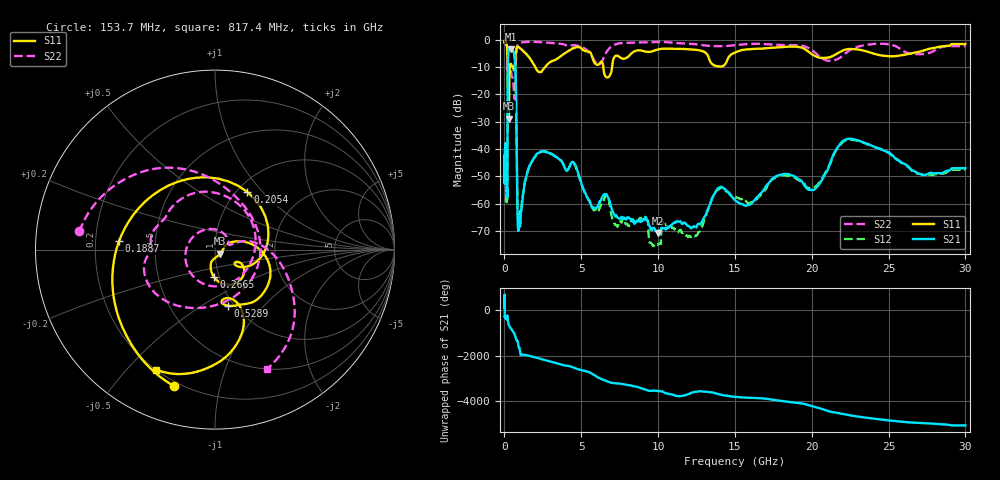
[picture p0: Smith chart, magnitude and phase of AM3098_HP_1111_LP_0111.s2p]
! Date/Time: Thu, Feb 28, 2019 8:47 AM
! Network Analyzer: Agilent Technologies E8364B Rev: A.07.50.67
! Sweep from 0.010 to 30.000 GHz, 1601 Points, Sweep Type: LOG
! Power Supply: 5.022 V, 0.002 A
# Hz S DB R 50
!freq MagS11 AngS11 MagS21 AngS21 MagS12 AngS12 MagS22 AngS22
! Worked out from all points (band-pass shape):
!   1601 points, 10 MHz to 30 GHz, reference 50 ohm
!   highest |S21| = -3.44 dB at 415.9 MHz (marker M1); lowest = -70.8 dB at 9.977 GHz (marker M2)
!   |S21| within 3 dB of the highest: 228.2 MHz to 665.6 MHz (437.4 MHz wide, 97.9 % of centre)
!   lowest |S11| = -28.9 dB at 290.1 MHz (marker M3), VSWR 1.07, Z = 52.8 - j2.4 ohm
!   |S11| at or under -10 dB: 210 MHz to 352 MHz (142 MHz wide, 50.5 % of centre); 2.009 GHz to 2.645 GHz (635.7 MHz wide, 27.3 % of centre); 6.433 GHz to 7.006 GHz (572.4 MHz wide, 8.52 % of centre)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
!   |S22| runs from -21.7 to -0.6 dB; largest |S21 - S12| = 0.014
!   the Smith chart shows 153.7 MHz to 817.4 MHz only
!   S11 on the Smith chart (normalised r, x): 153.7 MHz: 0.18, -0.73; 188.7 MHz: 0.30, +0.04; 205.4 MHz: 1.11, +0.83; 266.5 MHz: 0.94, -0.30; 528.9 MHz: 0.94, -0.65; 817.4 MHz: 0.20, -0.61
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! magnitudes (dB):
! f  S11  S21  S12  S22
! 10 MHz  -0.4  -44.0  -44.4  -0.6
! 38.04 MHz  -0.2  -41.4  -41.4  -0.7
! 106.1 MHz  -0.9  -40.9  -40.6  -1.4
! 144.7 MHz  -1.6  -54.6  -56.8  -2.0
! 153.7 MHz  -2.0  -56.1  -57.7  -2.4
! 188.7 MHz  -5.4  -52.7  -52.0  -9.3
! 205.4 MHz  -8.7  -23.4  -23.4  -9.7
! 266.5 MHz  -16.3  -4.0  -4.0  -8.8
! 290.1 MHz  -28.9  -3.6  -3.6  -9.4
! 415.9 MHz  -8.8  -3.4  -3.4  -10.8
! 528.9 MHz  -9.9  -3.9  -3.9  -13.9
! 550.5 MHz  -10.2  -4.1  -4.0  -14.6
! 714.1 MHz  -6.1  -10.8  -10.8  -12.9
! 817.4 MHz  -2.5  -51.0  -49.7  -2.8
! 921.7 MHz  -2.7  -68.5  -68.1  -1.4
! 2.084 GHz  -10.8  -41.9  -42.4  -0.8
! 4.48 GHz  -3.1  -44.9  -44.8  -2.0
! 7.926 GHz  -6.7  -65.9  -67.6  -1.1
! 9.977 GHz  -3.5  -70.8  -75.1  -0.8
! 20.1 GHz  -5.6  -55.1  -54.2  -4.1
! 22.56 GHz  -3.4  -36.3  -36.6  -3.5
! 30 GHz  -1.6  -47.1  -47.7  -2.3
